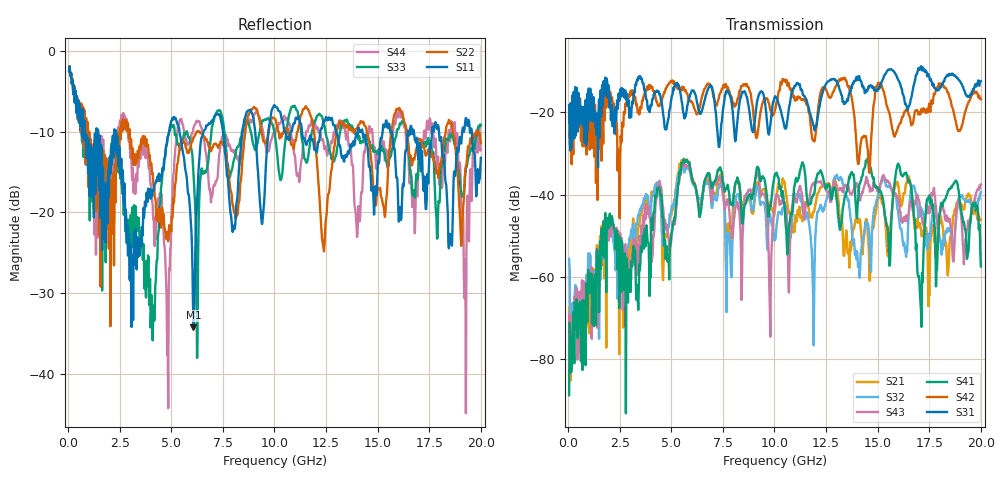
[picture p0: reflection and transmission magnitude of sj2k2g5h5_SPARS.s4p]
! FILE: E:\users\goganessyan\GBX_Backplane\FR408_backplane\1m_INBOUND_NEXT\sj2k2g5h5_SPARS.s4p
# MHZ S RI R 50.00
! FREQ  S11  S12  S13  S14
!  S21  S22  S23  S24
!  S31  S32  S33  S34
!  S41  S42  S43  S44
!  REAL  IMAG  REAL  IMAG  REAL  IMAG  REAL  IMAG
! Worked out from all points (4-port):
!   799 points, 50 MHz to 20 GHz, reference 50 ohm
!   strongest paths, dB at 50 MHz, 5.025 GHz, 10.03 GHz, 15.03 GHz, 20 GHz:
!     S31: -18.3, -16.0, -16.1, -14.4, -12.4
!     S42: -19.4, -12.5, -19.4, -12.8, -16.8
!     S41: -88.8, -49.2, -35.0, -38.3, -57.5
!     S43: -69.0, -48.4, -41.3, -39.0, -37.5
!     S32: -55.6, -42.7, -50.9, -40.0, -39.4
!     S21: -67.3, -44.2, -43.4, -40.9, -46.1
!   lowest |S11| = -34.2 dB at 6.075 GHz (marker M1), VSWR 1.04, Z = 52 + j0.27 ohm
!   |S11| at or under -10 dB: 2.327 GHz to 4.886 GHz (2.559 GHz wide, 71 % of centre); 5.397 GHz to 6.561 GHz (1.165 GHz wide, 19.5 % of centre); 17.97 GHz to 19.1 GHz (1.124 GHz wide, 6.07 % of centre)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
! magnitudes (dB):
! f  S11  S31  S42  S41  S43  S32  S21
! 50 MHz  -2.5  -18.3  -19.4  -88.8  -69.0  -55.6  -67.3
! 4.075 GHz  -18.0  -16.8  -13.8  -47.5  -55.3  -40.7  -40.1
! 4.8 GHz  -11.1  -23.1  -13.5  -54.6  -48.6  -49.1  -50.4
! 6.075 GHz  -34.2  -14.8  -18.4  -37.2  -37.3  -37.7  -36.7
! 9.175 GHz  -14.2  -16.9  -25.6  -33.2  -34.9  -37.9  -37.0
! 9.8 GHz  -8.4  -23.1  -19.5  -42.9  -74.5  -45.2  -42.1
! 20 GHz  -13.2  -12.4  -16.8  -57.5  -37.5  -39.4  -46.1
